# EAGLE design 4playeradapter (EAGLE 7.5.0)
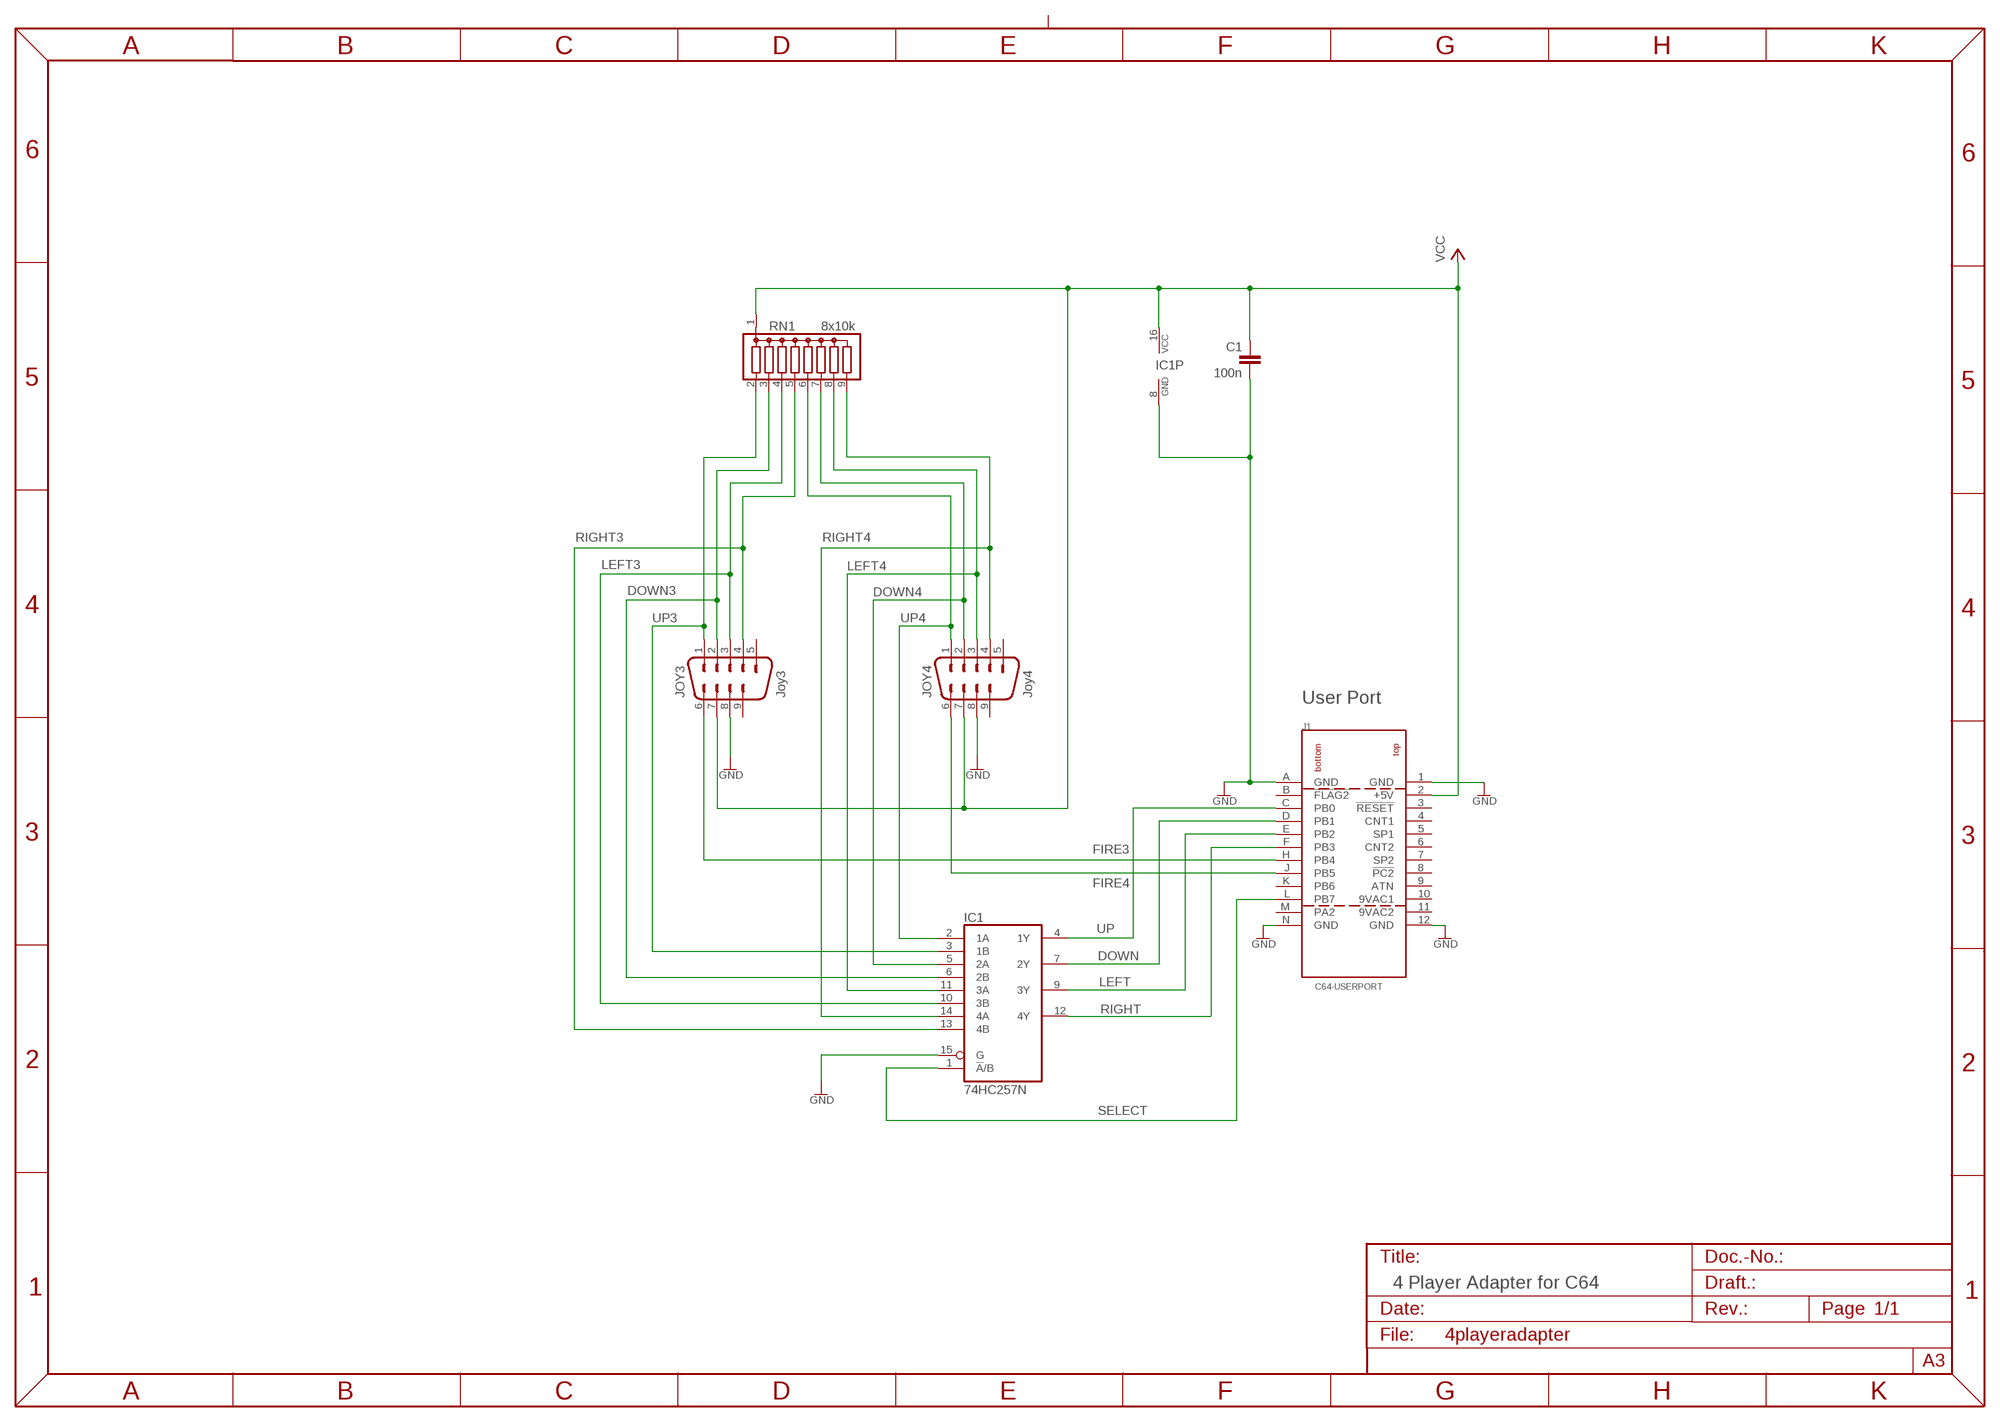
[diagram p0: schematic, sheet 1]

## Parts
C1  100n  C-EU050-024X044  [C050-024X044]
IC1  74HC257N  [DIL16]
J1  C64-USERPORT  [USERPORT]
JOY3  Joy3  M09D  [M09D]
JOY4  Joy4  M09D  [M09D]
RN1  8x10k  G08R  [SIL9]

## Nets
DOWN: IC1.7(2Y) J1.D(PB1)
DOWN3: IC1.6(2B) JOY3.2 RN1.3
DOWN4: IC1.5(2A) JOY4.2 RN1.7
FIRE3: J1.H(PB4) JOY3.6
FIRE4: J1.J(PB5) JOY4.6
GND: C1.2 IC1.8(GND) IC1.15(G) J1.1(GND) J1.12(GND) J1.A(GND) J1.N(GND) JOY3.8 JOY4.8
LEFT: IC1.9(3Y) J1.E(PB2)
LEFT3: IC1.10(3B) JOY3.3 RN1.4
LEFT4: IC1.11(3A) JOY4.3 RN1.8
RIGHT: IC1.12(4Y) J1.F(PB3)
RIGHT3: IC1.13(4B) JOY3.4 RN1.5
RIGHT4: IC1.14(4A) JOY4.4 RN1.9
SELECT: IC1.1(!A!/B) J1.L(PB7)
UP: IC1.4(1Y) J1.C(PB0)
UP3: IC1.3(1B) JOY3.1 RN1.2
UP4: IC1.2(1A) JOY4.1 RN1.6
VCC: C1.1 IC1.16(VCC) J1.2(+5V) JOY3.7 JOY4.7 RN1.1
Unconnected: J1.3(!RESET) J1.4(CNT1) J1.5(SP1) J1.6(CNT2) J1.7(SP2) J1.8(!PC2) J1.9(ATN) J1.B(!FLAG2) J1.K(PB6) J1.M(PA2) JOY3.5 JOY3.9 JOY4.5 JOY4.9

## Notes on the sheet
- User Port
- 4 Player Adapter for C64

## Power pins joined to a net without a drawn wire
9VAC1: J1.10(9VAC1)
9VAC2: J1.11(9VAC2)

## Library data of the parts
C1 = resistor:C-EU: CAPACITOR, European symbol
IC1 = 74xx-eu:74*257: Quadruple 2-to 1 line data SELECTOR/MULTIPLEXER
J1 = Commodore:C64-USERPORT
JOY3 JOY4 = con-subd:M09: SUB-D; OC_FARNELL: unknown; OC_NEWARK: unknown
RN1 = resistor-sil:G08R: SIL RESISTOR; OC_FARNELL: unknown; OC_NEWARK: unknown

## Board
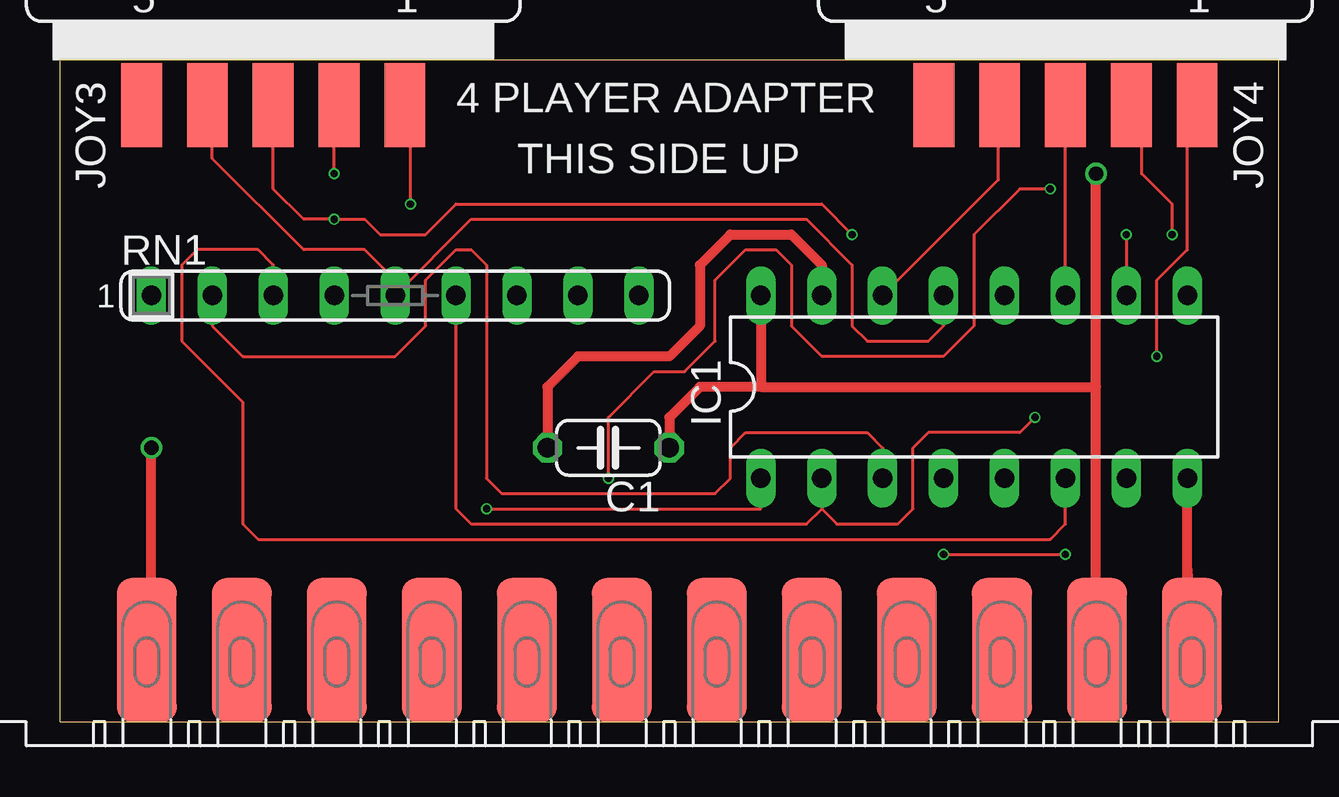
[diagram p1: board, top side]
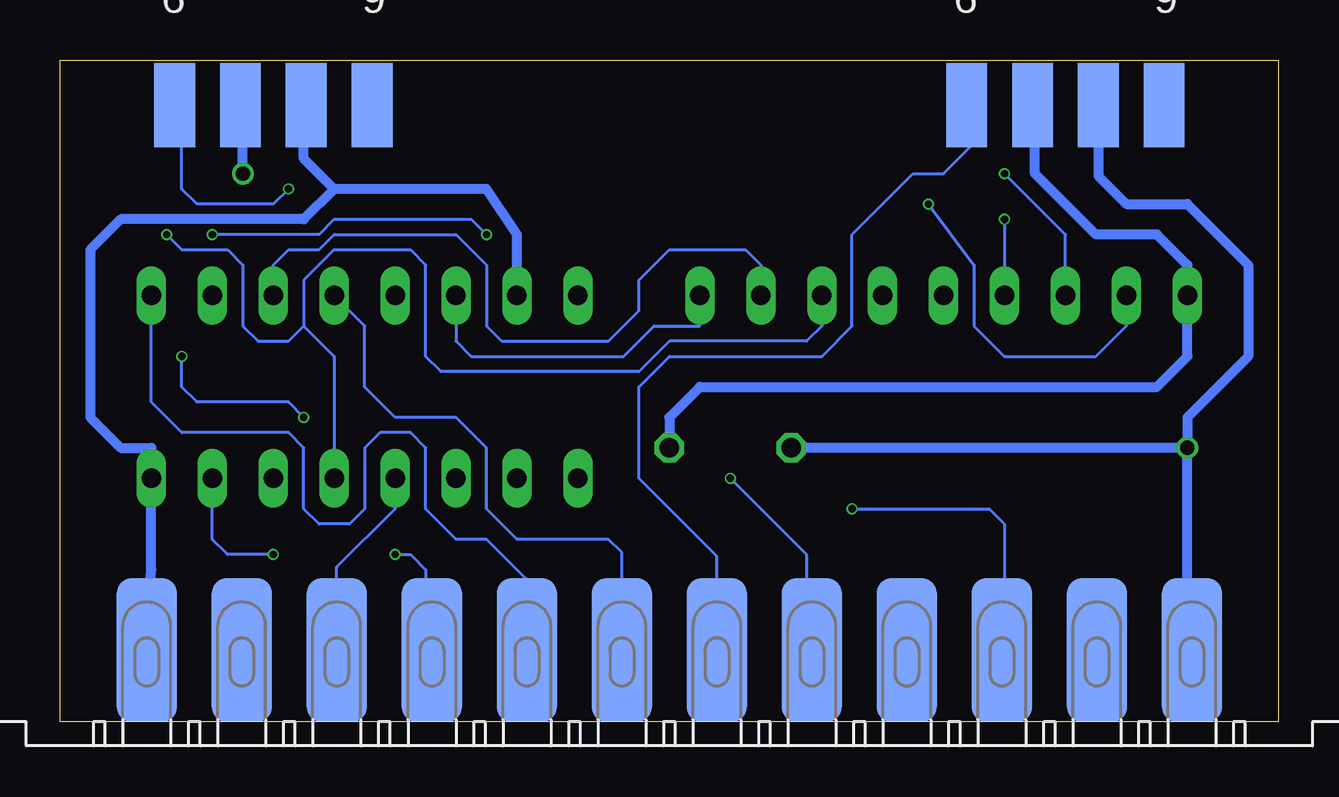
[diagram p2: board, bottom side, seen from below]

Size 50.8 x 27.6 mm. Coordinates in mm from the lower left corner, seen from the top.
Outline: 0,0 50.8,0 50.8,27.6 0,27.6 0,0
Copper layers (1*16): Top 0.035559375mm / dielectric 1.6mm / Bottom 0.035559375mm
Design rules "jlcpcb2layer *": minimum track width 5mil, minimum drill 12mil, track to track 5mil, track to pad 5mil, pad to pad 5mil, via to via 5mil, smd to smd 5mil, copper to edge 8mil, drill to drill 12mil, minimum pad ring 5mil, minimum via ring 3mil, stop-mask expansion 2.5mil, vias tented up to drill 0mil, thermal gap 10mil

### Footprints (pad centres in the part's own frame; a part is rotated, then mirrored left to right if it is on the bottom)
C050-024X044 = drill 0.813 octagon: 1 -2.54,0; 2 2.54,0
DIL16 = drill 0.813 long: 1 -8.89,-3.81; 2 -6.35,-3.81; 3 -3.81,-3.81; 4 -1.27,-3.81; 5 1.27,-3.81; 6 3.81,-3.81; 7 6.35,-3.81; 8 8.89,-3.81; 9 8.89,3.81; 10 6.35,3.81; 11 3.81,3.81; 12 1.27,3.81; 13 -1.27,3.81; 14 -3.81,3.81; 15 -6.35,3.81; 16 -8.89,3.81
USERPORT = smd 2.5 x 6: 1 -21.78,-3; 2 -17.82,-3; 3 -13.86,-3; 4 -9.9,-3; 5 -5.94,-3; 6 -1.98,-3; 7 1.98,-3; 8 5.94,-3; 9 9.9,-3; 10 13.86,-3; 11 17.82,-3; 12 21.78,-3 | smd 2.5 x 6 bottom: A -21.78,-3; B -17.82,-3; C -13.86,-3; D -9.9,-3; E -5.94,-3; F -1.98,-3; H 1.98,-3; J 5.94,-3; K 9.9,-3; L 13.86,-3; M 17.82,-3; N 21.78,-3
M09D = smd 1.7 x 3.5: 1 5.486,-6.045; 2 2.743,-6.045; 3 0,-6.045; 4 -2.743,-6.045; 5 -5.486,-6.045 | smd 1.7 x 3.5 bottom: 6 4.115,-6.045; 7 1.372,-6.045; 8 -1.372,-6.045; 9 -4.115,-6.045
SIL9 = drill 0.813 long: 1 -10.16,0; 2 -7.62,0; 3 -5.08,0; 4 -2.54,0; 5 0,0; 6 2.54,0; 7 5.08,0; 8 7.62,0; 9 10.16,0

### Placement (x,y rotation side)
C1  22.86,11.43 180 top
IC1  38.1,13.97 0 top
J1  25.4,0 180 top
JOY3  8.89,31.75 0 top
JOY4  41.91,31.75 0 top
RN1  13.97,17.78 0 top

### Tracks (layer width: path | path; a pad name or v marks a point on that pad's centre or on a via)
DOWN  (via drill 0.3, 0.3 pad 0.25)
  Top 0.127: v36.83,6.99 v41.91,6.99
  Bottom 0.127: 35.31,3.05 J1.D 35.56,5.71 35.56,6.35 36.2,6.99 v36.83,6.99 | v41.91,6.99 43.81,6.99 44.45,7.62 IC1.7
DOWN3  (via drill 0.3)
  Top 0.127: 11.56,25.65 JOY3.2 11.43,25.5 v11.43,22.86 | IC1.6 41.91,8.26 41.27,7.62 8.26,7.62 7.62,8.26 7.62,13.34 5.08,15.88 5.08,19.05 5.71,19.68 8.26,19.68 8.89,19.05 RN1.3
  Bottom 0.127: RN1.3 8.89,20.32 v11.43,22.86
DOWN4  (via drill 0.3)
  Top 0.127: 44.58,25.65 JOY4.2 45.09,25.27 45.09,22.86 46.35,21.59 v46.35,20.32
  Bottom 0.127: v46.35,20.32 45.72,19.68 43.81,19.68 43.18,19.05 43.18,16.51 42.55,15.88 41.27,15.88 40.64,16.51 | RN1.7 19.05,16.51 19.68,15.88 25.4,15.88 26.67,14.61 34.92,14.61 35.56,15.24 35.56,19.05 36.2,19.68 39.37,19.68 40.64,18.41 40.64,16.51 | 40.64,16.51 39.37,15.24 IC1.5
FIRE3
  Bottom 0.127: J1.H 23.42,6.91 26.67,10.16 26.67,13.97 25.4,15.24 19.05,15.24 17.78,16.51 17.78,20.32 15.24,22.86 13.97,22.86 12.7,24.13 12.7,26.01 | 12.7,25.4 JOY3.6 12.7,26.01 | 12.7,26.67 12.7,26.01
FIRE4  (via drill 0.3)
  Top 0.127: v22.86,10.16 22.86,12.7 24.77,14.61 26.04,14.61 27.3,15.88 27.3,18.41 28.57,19.68 29.84,19.68 30.48,19.05 30.48,16.51 31.75,15.24 36.83,15.24 38.1,16.51 38.1,20.32 40.01,22.23 v41.27,22.23
  Bottom 0.127: 20.57,4.06 19.56,3.05 J1.J | 45.97,25.65 JOY4.6 45.72,25.4 45.72,22.23 45.09,21.59 41.91,21.59 v41.27,22.23 | 19.05,3.41 J1.J | v22.86,10.16 19.68,6.99 19.68,5.71 J1.J
GND  (via drill 0.6)
  Top 0.406: IC1.15 31.75,19.05 30.48,20.32 27.94,20.32 26.67,19.05 26.67,16.51 25.4,15.24 21.59,15.24 20.32,13.97 C1.2 | 3.62,4 3.81,5.08 | J1.12 3.62,4 | 3.62,4 3.81,3.81 3.81,5.08 | 3.81,5.08 v3.81,11.43 | 46.99,5.08 46.99,5.27 47.18,5.27 J1.1 46.99,6.35 IC1.8 46.99,3.81
  Bottom 0.406: J1.1 46.99,6.35 IC1.8 46.99,11.43 48.26,11.43 49.53,12.7 49.53,19.68 48.26,20.95 40.64,20.95 39.37,22.23 | IC1.15 31.75,20.32 33.02,22.23 39.37,22.23 | 39.37,22.23 40.64,23.5 40.64,25.6 JOY4.8 | J1.12 3.81,3 v3.81,11.43 | JOY3.8 7.52,22.76 6.35,21.59 3.81,21.59 1.27,19.05 1.27,15.24 3.81,12.7 v3.81,11.43 | v3.81,11.43 C1.2
LEFT
  Bottom 0.127: J1.E 31.37,3.05 31.37,5.97 33.02,7.62 34.29,7.62 35.56,8.89 35.56,11.43 36.2,12.06 37.47,12.06 38.1,11.43 38.1,8.89 38.73,8.26 40.01,8.26 40.64,8.89 40.64,11.43 41.27,12.06 45.72,12.06 46.99,13.34 IC1.9
LEFT3  (via drill 0.3)
  Top 0.127: v44.45,20.32 IC1.10 | v33.02,20.32 31.75,21.59 16.51,21.59 15.24,20.32 13.34,20.32 12.7,20.95 v11.43,20.95 10.16,20.95 8.89,22.23 JOY3.3
  Bottom 0.127: v11.43,20.95 RN1.4 | v44.45,20.32 40.01,20.32 39.37,20.95 33.66,20.95 v33.02,20.32
LEFT4
  Top 0.127: IC1.11 JOY4.3
  Bottom 0.127: IC1.11 41.91,19.05 41.27,19.68 40.01,19.68 39.37,20.32 34.29,20.32 33.02,19.05 33.02,16.51 32.38,15.88 27.94,15.88 26.67,17.14 26.67,18.41 25.4,19.68 22.23,19.68 21.59,19.05 RN1.8
RIGHT
  Bottom 0.127: J1.F 27.38,7.06 27.94,7.62 31.75,7.62 33.02,8.89 33.02,11.43 34.29,12.7 36.83,12.7 38.1,13.97 38.1,16.51 IC1.12
RIGHT3
  Top 0.127: IC1.13 36.83,16.51 36.2,15.88 33.66,15.88 33.02,16.51 33.02,19.05 31.11,20.95 17.14,20.95 RN1.5 13.97,18.41 12.7,19.68 10.16,19.68 6.35,23.5 6.35,25.5 JOY3.4
RIGHT4
  Top 0.127: IC1.14 39.12,22.61 39.12,25.65 JOY4.4
  Bottom 0.127: IC1.14 34.29,15.88 33.66,15.24 27.3,15.24 26.04,16.51 24.13,16.51 RN1.9
SELECT  (via drill 0.3)
  Top 0.127: v17.78,8.89 29.21,8.89 IC1.1
  Bottom 0.127: 11.56,3.3 11.56,3.05 J1.L | 11.43,3.11 J1.L | v17.78,8.89 12.06,8.89 11.43,8.26 11.43,5.71 J1.L
UP
  Bottom 0.127: J1.C 39.26,6.46 36.83,8.89 IC1.4
UP3  (via drill 0.3)
  Top 0.127: 14.35,25.65 JOY3.1 14.61,25.48 v14.61,21.59 | RN1.2 6.35,16.51 7.62,15.24 13.97,15.24 15.24,16.51 15.24,18.41 16.51,19.68 17.14,19.68 17.78,19.05 17.78,10.16 18.41,9.53 27.3,9.53 27.94,10.16 27.94,11.43 28.57,12.06 33.66,12.06 34.29,11.43 IC1.3
  Bottom 0.127: v14.61,21.59 12.7,19.05 12.7,16.51 11.43,15.24 7.62,15.24 6.35,16.51 RN1.2
UP4  (via drill 0.3)
  Top 0.127: 47.37,25.65 JOY4.1 46.99,24.13 46.99,19.68 45.72,18.41 v45.72,15.24 | IC1.2 31.75,8.89 | 31.75,8.89 32.38,8.26 34.92,8.26 35.56,8.89 35.56,11.43 36.2,12.06 40.01,12.06 v40.64,12.7 | RN1.6 16.51,8.89 17.14,8.26 31.11,8.26 31.75,8.89
  Bottom 0.127: v40.64,12.7 41.27,13.34 45.09,13.34 45.72,13.97 v45.72,15.24
VCC  (via drill 0.6)
  Top 0.406: J1.2 43.18,3 43.18,13.97 | 43.18,13.97 v43.18,22.86 | IC1.16 29.21,13.97 | 29.21,13.97 43.18,13.97 | 29.21,13.97 26.67,13.97 25.4,12.7 C1.1
  Bottom 0.406: JOY3.7 10.16,25.6 10.16,22.86 7.62,20.32 5.08,20.32 3.81,19.05 RN1.1 3.81,15.24 5.08,13.97 24.13,13.97 25.4,12.7 C1.1 | v43.18,22.86 43.18,24.13 43.28,24.13 JOY4.7

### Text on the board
tNames: 4 PLAYER ADAPTER | THIS SIDE UP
